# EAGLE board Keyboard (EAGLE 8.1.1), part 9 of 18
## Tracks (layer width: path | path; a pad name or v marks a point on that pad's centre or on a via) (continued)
S$8799 (continued)
  Bottom 0: 282.46,76.14 282.5,76.06
S$8800
  Bottom 0: 282.5,76.06 282.55,76.01
S$8801
  Bottom 0: 282.55,76.01 282.62,75.97
S$8802
  Bottom 0: 282.62,75.97 282.7,75.96
S$8803
  Bottom 0: 282.7,75.96 284.86,75.96
S$8804
  Bottom 0: 284.86,75.96 284.94,75.97
S$8805
  Bottom 0: 284.94,75.97 285.01,76.01
S$8806
  Bottom 0: 285.01,76.01 285.06,76.06
S$8807
  Bottom 0: 285.06,76.06 285.1,76.14
S$8808
  Bottom 0: 285.1,76.14 285.11,76.21
S$8809
  Bottom 0: 285.11,76.21 285.11,77.41
S$8810
  Bottom 0: 285.11,77.41 285.1,77.49
S$8811
  Bottom 0: 285.1,77.49 285.06,77.56
S$8812
  Bottom 0: 285.06,77.56 285.01,77.61
S$8813
  Bottom 0: 285.01,77.61 284.94,77.66
S$8814
  Bottom 0: 284.94,77.66 284.86,77.67
S$8815
  Bottom 0: 284.86,77.67 282.76,77.67
S$8816
  Bottom 0: 282.76,77.67 282.76,77.97
S$8817
  Bottom 0: 282.76,77.97 284.86,77.97
S$8818
  Bottom 0: 284.86,77.97 284.94,77.97
S$8819
  Bottom 0: 284.94,77.97 285.01,78.02
S$8820
  Bottom 0: 285.01,78.02 285.06,78.07
S$8821
  Bottom 0: 285.06,78.07 285.1,78.14
S$8822
  Bottom 0: 285.1,78.14 285.11,78.22
S$8823
  Bottom 0: 285.11,78.22 285.11,79.42
S$8824
  Bottom 0: 285.11,79.42 285.1,79.49
S$8825
  Bottom 0: 285.1,79.49 285.06,79.57
S$8826
  Bottom 0: 285.06,79.57 285.01,79.62
S$8827
  Bottom 0: 285.01,79.62 284.94,79.66
S$8828
  Bottom 0: 284.94,79.66 284.86,79.67
S$8829
  Bottom 0: 284.86,79.67 282.76,79.67
S$8830
  Bottom 0: 282.76,79.67 282.76,79.97
S$8831
  Bottom 0: 282.76,79.97 284.86,79.97
S$8832
  Bottom 0: 284.86,79.97 284.94,79.98
S$8833
  Bottom 0: 284.94,79.98 285.01,80.02
S$8834
  Bottom 0: 285.01,80.02 285.06,80.08
S$8835
  Bottom 0: 285.06,80.08 285.1,80.15
S$8836
  Bottom 0: 285.1,80.15 285.11,80.23
S$8837
  Bottom 0: 285.11,80.23 285.11,81.42
S$8838
  Bottom 0: 285.11,81.42 285.1,81.5
S$8839
  Bottom 0: 285.1,81.5 285.1,81.51
S$8840
  Bottom 0: 285.1,81.51 286.16,82.57
S$8841
  Bottom 0: 286.16,82.57 286.43,82.59
S$8842
  Bottom 0: 286.43,82.59 286.69,82.7
S$8843
  Bottom 0: 286.69,82.7 286.9,82.9
S$8844
  Bottom 0: 286.9,82.9 287.03,83.14
S$8845
  Bottom 0: 287.03,83.14 287.07,83.42
S$8846
  Bottom 0: 287.07,83.42 287.03,83.7
S$8847
  Bottom 0: 287.03,83.7 286.99,83.77
S$8848
  Bottom 0: 286.99,83.77 287.05,83.78
S$8849
  Bottom 0: 287.05,83.78 287.03,83.72
S$8850
  Bottom 0: 287.03,83.72 287.52,83.72
S$8851
  Bottom 0: 287.52,83.72 287.52,83.94
S$8852
  Bottom 0: 287.52,83.94 287.68,84.09
S$8853
  Bottom 0: 287.68,84.09 287.81,84.34
S$8854
  Bottom 0: 287.81,84.34 287.86,84.61
S$8855
  Bottom 0: 287.86,84.61 287.81,84.89
S$8856
  Bottom 0: 287.81,84.89 287.68,85.14
S$8857
  Bottom 0: 287.68,85.14 287.48,85.33
S$8858
  Bottom 0: 287.48,85.33 287.22,85.44
S$8859
  Bottom 0: 287.22,85.44 286.94,85.46
S$8860
  Bottom 0: 286.94,85.46 286.66,85.4
S$8861
  Bottom 0: 286.66,85.4 286.43,85.25
S$8862
  Bottom 0: 286.43,85.25 286.25,85.02
S$8863
  Bottom 0: 286.25,85.02 286.22,84.92
S$8864
  Bottom 0: 286.22,84.92 286.11,85.14
S$8865
  Bottom 0: 286.11,85.14 285.9,85.33
S$8866
  Bottom 0: 285.9,85.33 285.64,85.44
S$8867
  Bottom 0: 285.64,85.44 285.36,85.46
S$8868
  Bottom 0: 285.36,85.46 285.16,85.41
S$8869
  Bottom 0: 285.16,85.41 288.85,89.1
S$8870
  Bottom 0: 288.85,89.1 289.3,89.1
S$8871
  Bottom 0: 289.3,89.1 289.3,89.56
S$8872
  Bottom 0: 289.3,89.56 289.38,89.64
S$8873
  Bottom 0: 289.38,89.64 290.45,89.64
S$8874
  Bottom 0: 290.45,89.64 290.45,89.1
S$8875
  Bottom 0: 290.45,89.1 291.15,89.1
S$8876
  Bottom 0: 291.15,89.1 291.1,89.2
S$8877
  Bottom 0: 291.1,89.2 290.9,89.49
S$8878
  Bottom 0: 290.9,89.49 290.72,89.64
S$8879
  Bottom 0: 290.72,89.64 293.99,89.64
S$8880
  Bottom 0: 293.99,89.64 293.99,82.85
S$8881
  Bottom 0: 293.99,82.85 294,82.76
S$8882
  Bottom 0: 294,82.76 294.02,82.67
S$8883
  Bottom 0: 294.02,82.67 294.05,82.59
S$8884
  Bottom 0: 294.05,82.59 294.1,82.51
S$8885
  Bottom 0: 294.1,82.51 294.16,82.45
S$8886
  Bottom 0: 294.16,82.45 298.75,77.85
S$8887
  Bottom 0: 298.75,77.85 298.75,70.75
S$8888
  Bottom 0: 298.75,70.75 298.63,70.78
S$8889
  Bottom 0: 298.63,70.78 298.33,70.76
S$8890
  Bottom 0: 298.33,70.76 298.05,70.65
S$8891
  Bottom 0: 298.05,70.65 297.81,70.46
S$8892
  Bottom 0: 297.81,70.46 297.8,70.44
S$8893
  Bottom 0: 297.8,70.44 297.8,70.66
S$8894
  Bottom 0: 297.8,70.66 297.79,70.74
S$8895
  Bottom 0: 297.79,70.74 297.75,70.81
S$8896
  Bottom 0: 297.75,70.81 297.69,70.86
S$8897
  Bottom 0: 297.69,70.86 297.62,70.9
S$8898
  Bottom 0: 297.62,70.9 297.54,70.91
S$8899
  Bottom 0: 297.54,70.91 296.47,70.91
S$8900
  Bottom 0: 296.47,70.91 296.47,71.04
S$8901
  Bottom 0: 296.47,71.04 296.45,71.1
S$8902
  Bottom 0: 296.45,71.1 296.45,71.16
S$8903
  Bottom 0: 296.45,71.16 296.42,71.21
S$8904
  Bottom 0: 296.42,71.21 296.4,71.26
S$8905
  Bottom 0: 296.4,71.26 296.38,71.3
S$8906
  Bottom 0: 296.38,71.3 296.34,71.36
S$8907
  Bottom 0: 296.34,71.36 295.29,72.4
S$8908
  Bottom 0: 295.29,72.4 295.31,72.42
S$8909
  Bottom 0: 295.31,72.42 295.44,72.72
S$8910
  Bottom 0: 295.44,72.72 295.49,73.04
S$8911
  Bottom 0: 295.49,73.04 295.44,73.36
S$8912
  Bottom 0: 295.44,73.36 295.31,73.66
S$8913
  Bottom 0: 295.31,73.66 295.11,73.92
S$8914
  Bottom 0: 295.11,73.92 294.84,74.11
S$8915
  Bottom 0: 294.84,74.11 294.53,74.21
S$8916
  Bottom 0: 294.53,74.21 294.21,74.23
S$8917
  Bottom 0: 294.21,74.23 293.89,74.17
S$8918
  Bottom 0: 293.89,74.17 293.6,74.02
S$8919
  Bottom 0: 293.6,74.02 293.38,73.8
S$8920
  Bottom 0: 293.38,73.8 293.38,73.89
S$8921
  Bottom 0: 293.38,73.89 293.82,74.33
S$8922
  Bottom 0: 293.82,74.33 293.89,74.3
S$8923
  Bottom 0: 293.89,74.3 294.21,74.23
S$8924
  Bottom 0: 294.21,74.23 294.53,74.25
S$8925
  Bottom 0: 294.53,74.25 294.84,74.36
S$8926
  Bottom 0: 294.84,74.36 295.11,74.55
S$8927
  Bottom 0: 295.11,74.55 295.31,74.8
S$8928
  Bottom 0: 295.31,74.8 295.44,75.1
S$8929
  Bottom 0: 295.44,75.1 295.49,75.42
S$8930
  Bottom 0: 295.49,75.42 295.44,75.74
S$8931
  Bottom 0: 295.44,75.74 295.31,76.04
S$8932
  Bottom 0: 295.31,76.04 295.11,76.29
S$8933
  Bottom 0: 295.11,76.29 294.84,76.48
S$8934
  Bottom 0: 294.84,76.48 294.53,76.59
S$8935
  Bottom 0: 294.53,76.59 294.21,76.61
S$8936
  Bottom 0: 294.21,76.61 293.9,76.54
S$8937
  Bottom 0: 293.9,76.54 294.04,76.69
S$8938
  Bottom 0: 294.04,76.69 297,76.69
S$8939
  Bottom 0: 297,76.69 297.07,76.69
S$8940
  Bottom 0: 297.07,76.69 297.14,76.7
S$8941
  Bottom 0: 297.14,76.7 297.2,76.73
S$8942
  Bottom 0: 297.2,76.73 297.26,76.77
S$8943
  Bottom 0: 297.26,76.77 297.32,76.81
S$8944
  Bottom 0: 297.32,76.81 297.53,77.03
S$8945
  Bottom 0: 297.53,77.03 297.63,77.02
S$8946
  Bottom 0: 297.63,77.02 297.88,77.08
S$8947
  Bottom 0: 297.88,77.08 298.08,77.23
S$8948
  Bottom 0: 298.08,77.23 298.21,77.45
S$8949
  Bottom 0: 298.21,77.45 298.26,77.7
S$8950
  Bottom 0: 298.26,77.7 298.21,77.94
S$8951
  Bottom 0: 298.21,77.94 298.08,78.16
S$8952
  Bottom 0: 298.08,78.16 297.88,78.31
S$8953
  Bottom 0: 297.88,78.31 297.63,78.38
S$8954
  Bottom 0: 297.63,78.38 297.39,78.36
S$8955
  Bottom 0: 297.39,78.36 297.16,78.25
S$8956
  Bottom 0: 297.16,78.25 296.99,78.06
S$8957
  Bottom 0: 296.99,78.06 296.9,77.82
S$8958
  Bottom 0: 296.9,77.82 296.9,77.65
S$8959
  Bottom 0: 296.9,77.65 296.82,77.57
S$8960
  Bottom 0: 296.82,77.57 296.36,77.57
S$8961
  Bottom 0: 296.36,77.57 296.53,77.71
S$8962
  Bottom 0: 296.53,77.71 296.74,77.99
S$8963
  Bottom 0: 296.74,77.99 296.86,78.32
S$8964
  Bottom 0: 296.86,78.32 296.91,78.66
S$8965
  Bottom 0: 296.91,78.66 296.86,79.01
S$8966
  Bottom 0: 296.86,79.01 296.74,79.33
S$8967
  Bottom 0: 296.74,79.33 296.53,79.62
S$8968
  Bottom 0: 296.53,79.62 296.25,79.84
S$8969
  Bottom 0: 296.25,79.84 295.94,79.99
S$8970
  Bottom 0: 295.94,79.99 295.6,80.05
S$8971
  Bottom 0: 295.6,80.05 295.25,80.03
S$8972
  Bottom 0: 295.25,80.03 295.14,80
S$8973
  Bottom 0: 295.14,80 294.84,80.05
S$8974
  Bottom 0: 294.84,80.05 294.49,80.03
S$8975
  Bottom 0: 294.49,80.03 294.15,79.93
S$8976
  Bottom 0: 294.15,79.93 293.86,79.74
S$8977
  Bottom 0: 293.86,79.74 293.62,79.48
S$8978
  Bottom 0: 293.62,79.48 293.45,79.17
S$8979
  Bottom 0: 293.45,79.17 293.43,79.1
S$8980
  Bottom 0: 293.43,79.1 293,79.1
S$8981
  Bottom 0: 293,79.1 292.93,79.1
S$8982
  Bottom 0: 292.93,79.1 292.87,79.08
S$8983
  Bottom 0: 292.87,79.08 292.8,79.06
S$8984
  Bottom 0: 292.8,79.06 292.74,79.02
S$8985
  Bottom 0: 292.74,79.02 292.69,78.98
S$8986
  Bottom 0: 292.69,78.98 287.71,74
S$8987
  Bottom 0: 287.71,74 287.46,74.05
S$8988
  Bottom 0: 287.46,74.05 287.15,74.03
S$8989
  Bottom 0: 287.15,74.03 286.88,73.92
S$8990
  Bottom 0: 286.88,73.92 286.69,73.78
S$8991
  Bottom 0: 286.69,73.78 286.69,79.34
S$8992
  Bottom 0: 286.69,79.34 287.06,79.71
S$8993
  Bottom 0: 287.06,79.71 287.15,79.67
S$8994
  Bottom 0: 287.15,79.67 287.46,79.65
S$8995
  Bottom 0: 287.46,79.65 287.75,79.72
S$8996
  Bottom 0: 287.75,79.72 288.02,79.87
S$8997
  Bottom 0: 288.02,79.87 288.22,80.09
S$8998
  Bottom 0: 288.22,80.09 288.35,80.36
S$8999
  Bottom 0: 288.35,80.36 288.4,80.66
S$9000
  Bottom 0: 288.4,80.66 288.35,80.96
S$9001
  Bottom 0: 288.35,80.96 288.22,81.24
S$9002
  Bottom 0: 288.22,81.24 288.02,81.45
S$9003
  Bottom 0: 288.02,81.45 287.75,81.61
S$9004
  Bottom 0: 287.75,81.61 287.46,81.67
S$9005
  Bottom 0: 287.46,81.67 287.15,81.65
S$9006
  Bottom 0: 287.15,81.65 286.88,81.54
S$9007
  Bottom 0: 286.88,81.54 286.64,81.35
S$9008
  Bottom 0: 286.64,81.35 286.47,81.11
S$9009
  Bottom 0: 286.47,81.11 286.38,80.81
S$9010
  Bottom 0: 286.38,80.81 286.38,80.51
S$9011
  Bottom 0: 286.38,80.51 286.43,80.34
S$9012
  Bottom 0: 286.43,80.34 285.94,79.84
S$9013
  Bottom 0: 285.94,79.84 285.89,79.79
S$9014
  Bottom 0: 285.89,79.79 285.85,79.73
S$9015
  Bottom 0: 285.85,79.73 285.83,79.67
S$9016
  Bottom 0: 285.83,79.67 285.81,79.6
S$9017
  Bottom 0: 285.81,79.6 285.81,79.53
S$9018
  Bottom 0: 285.81,79.53 285.81,65.56
S$9019
  Bottom 0: 285.81,65.56 285.32,65.07
S$9020
  Bottom 0: 285.32,65.07 285.09,65.05
S$9021
  Bottom 0: 285.09,65.05 284.86,64.94
S$9022
  Bottom 0: 284.86,64.94 284.69,64.75
S$9023
  Bottom 0: 284.69,64.75 284.6,64.52
S$9024
  Bottom 0: 284.6,64.52 284.6,64.27
S$9025
  Bottom 0: 284.6,64.27 284.69,64.03
S$9026
  Bottom 0: 284.69,64.03 284.86,63.84
S$9027
  Bottom 0: 284.86,63.84 285.09,63.73
S$9028
  Bottom 0: 285.09,63.73 285.33,63.71
S$9029
  Bottom 0: 285.33,63.71 285.58,63.78
S$9030
  Bottom 0: 285.58,63.78 285.78,63.93
S$9031
  Bottom 0: 285.78,63.93 285.92,64.14
S$9032
  Bottom 0: 285.92,64.14 285.96,64.39
S$9033
  Bottom 0: 285.96,64.39 285.95,64.45
S$9034
  Bottom 0: 285.95,64.45 286.56,65.06
S$9035
  Bottom 0: 286.56,65.06 286.6,65.12
S$9036
  Bottom 0: 286.6,65.12 286.65,65.18
S$9037
  Bottom 0: 286.65,65.18 286.67,65.24
S$9038
  Bottom 0: 286.67,65.24 286.69,65.31
S$9039
  Bottom 0: 286.69,65.31 286.69,65.38
S$9040
  Bottom 0: 286.69,65.38 286.69,72.3
S$9041
  Bottom 0: 286.69,72.3 286.88,72.16
S$9042
  Bottom 0: 286.88,72.16 287.15,72.05
S$9043
  Bottom 0: 287.15,72.05 287.46,72.03
S$9044
  Bottom 0: 287.46,72.03 287.75,72.1
S$9045
  Bottom 0: 287.75,72.1 288.02,72.25
S$9046
  Bottom 0: 288.02,72.25 288.22,72.47
S$9047
  Bottom 0: 288.22,72.47 288.35,72.74
S$9048
  Bottom 0: 288.35,72.74 288.4,73.04
S$9049
  Bottom 0: 288.4,73.04 288.35,73.34
S$9050
  Bottom 0: 288.35,73.34 288.34,73.37
S$9051
  Bottom 0: 288.34,73.37 293.19,78.22
S$9052
  Bottom 0: 293.19,78.22 293.43,78.22
S$9053
  Bottom 0: 293.43,78.22 293.45,78.15
S$9054
  Bottom 0: 293.45,78.15 293.62,77.84
S$9055
  Bottom 0: 293.62,77.84 293.86,77.58
S$9056
  Bottom 0: 293.86,77.58 293.89,77.57
S$9057
  Bottom 0: 293.89,77.57 293.85,77.57
S$9058
  Bottom 0: 293.85,77.57 293.78,77.56
S$9059
  Bottom 0: 293.78,77.56 293.71,77.55
S$9060
  Bottom 0: 293.71,77.55 293.65,77.52
S$9061
  Bottom 0: 293.65,77.52 293.59,77.48
S$9062
  Bottom 0: 293.59,77.48 293.54,77.44
S$9063
  Bottom 0: 293.54,77.44 290.09,74
S$9064
  Bottom 0: 290.09,74 289.84,74.05
S$9065
  Bottom 0: 289.84,74.05 289.54,74.03
S$9066
  Bottom 0: 289.54,74.03 289.26,73.92
S$9067
  Bottom 0: 289.26,73.92 289.02,73.73
S$9068
  Bottom 0: 289.02,73.73 288.85,73.48
S$9069
  Bottom 0: 288.85,73.48 288.76,73.19
S$9070
  Bottom 0: 288.76,73.19 288.76,72.89
S$9071
  Bottom 0: 288.76,72.89 288.85,72.6
S$9072
  Bottom 0: 288.85,72.6 289.02,72.35
S$9073
  Bottom 0: 289.02,72.35 289.26,72.16
S$9074
  Bottom 0: 289.26,72.16 289.54,72.05
S$9075
  Bottom 0: 289.54,72.05 289.84,72.03
S$9076
  Bottom 0: 289.84,72.03 290.14,72.1
S$9077
  Bottom 0: 290.14,72.1 290.4,72.25
S$9078
  Bottom 0: 290.4,72.25 290.6,72.47
S$9079
  Bottom 0: 290.6,72.47 290.74,72.74
S$9080
  Bottom 0: 290.74,72.74 290.78,73.04
S$9081
  Bottom 0: 290.78,73.04 290.74,73.34
S$9082
  Bottom 0: 290.74,73.34 290.72,73.37
S$9083
  Bottom 0: 290.72,73.37 293.17,75.82
S$9084
  Bottom 0: 293.17,75.82 293.11,75.58
S$9085
  Bottom 0: 293.11,75.58 293.11,75.26
S$9086
  Bottom 0: 293.11,75.26 293.19,74.94
S$9087
  Bottom 0: 293.19,74.94 292.63,74.38
S$9088
  Bottom 0: 292.63,74.38 292.58,74.33
S$9089
  Bottom 0: 292.58,74.33 292.55,74.27
S$9090
  Bottom 0: 292.55,74.27 292.51,74.21
S$9091
  Bottom 0: 292.51,74.21 292.5,74.14
S$9092
  Bottom 0: 292.5,74.14 292.49,74.07
S$9093
  Bottom 0: 292.49,74.07 292.49,70.52
S$9094
  Bottom 0: 292.49,70.52 292.5,70.45
S$9095
  Bottom 0: 292.5,70.45 292.51,70.38
S$9096
  Bottom 0: 292.51,70.38 292.54,70.32
S$9097
  Bottom 0: 292.54,70.32 292.58,70.26
S$9098
  Bottom 0: 292.58,70.26 292.62,70.2
S$9099
  Bottom 0: 292.62,70.2 294.75,68.08
S$9100
  Bottom 0: 294.75,68.08 294.81,68.03
S$9101
  Bottom 0: 294.81,68.03 294.87,67.99
S$9102
  Bottom 0: 294.87,67.99 294.93,67.97
S$9103
  Bottom 0: 294.93,67.97 294.99,67.95
S$9104
  Bottom 0: 294.99,67.95 295.06,67.95
S$9105
  Bottom 0: 295.06,67.95 299.75,67.95
S$9106
  Bottom 0: 299.75,67.95 299.82,67.95
S$9107
  Bottom 0: 299.82,67.95 299.89,67.97
S$9108
  Bottom 0: 299.89,67.97 299.95,67.99
S$9109
  Bottom 0: 299.95,67.99 300.01,68.03
S$9110
  Bottom 0: 300.01,68.03 300.06,68.08
S$9111
  Bottom 0: 300.06,68.08 300.91,68.91
S$9112
  Bottom 0: 300.91,68.91 300.95,68.97
S$9113
  Bottom 0: 300.95,68.97 300.99,69.03
S$9114
  Bottom 0: 300.99,69.03 301.01,69.09
S$9115
  Bottom 0: 301.01,69.09 301.03,69.16
S$9116
  Bottom 0: 301.03,69.16 301.03,69.22
S$9117
  Bottom 0: 301.03,69.22 301.03,72.25
S$9118
  Bottom 0: 301.03,72.25 301.22,72.07
S$9119
  Bottom 0: 301.22,72.07 301.51,71.92
S$9120
  Bottom 0: 301.51,71.92 301.83,71.85
S$9121
  Bottom 0: 301.83,71.85 302.15,71.87
S$9122
  Bottom 0: 302.15,71.87 302.46,71.98
S$9123
  Bottom 0: 302.46,71.98 302.73,72.17
S$9124
  Bottom 0: 302.73,72.17 302.93,72.42
S$9125
  Bottom 0: 302.93,72.42 303.06,72.72
S$9126
  Bottom 0: 303.06,72.72 303.11,73.04
S$9127
  Bottom 0: 303.11,73.04 303.06,73.36
S$9128
  Bottom 0: 303.06,73.36 302.93,73.66
S$9129
  Bottom 0: 302.93,73.66 302.73,73.92
S$9130
  Bottom 0: 302.73,73.92 302.48,74.09
S$9131
  Bottom 0: 302.48,74.09 302.48,74.37
S$9132
  Bottom 0: 302.48,74.37 302.73,74.55
S$9133
  Bottom 0: 302.73,74.55 302.93,74.8
S$9134
  Bottom 0: 302.93,74.8 303.06,75.1
S$9135
  Bottom 0: 303.06,75.1 303.11,75.42
S$9136
  Bottom 0: 303.11,75.42 303.06,75.74
S$9137
  Bottom 0: 303.06,75.74 302.93,76.04
S$9138
  Bottom 0: 302.93,76.04 302.73,76.29
S$9139
  Bottom 0: 302.73,76.29 302.46,76.48
S$9140
  Bottom 0: 302.46,76.48 302.15,76.59
S$9141
  Bottom 0: 302.15,76.59 301.83,76.61
S$9142
  Bottom 0: 301.83,76.61 301.51,76.54
S$9143
  Bottom 0: 301.51,76.54 301.22,76.4
S$9144
  Bottom 0: 301.22,76.4 301.03,76.22
S$9145
  Bottom 0: 301.03,76.22 301.03,78.99
S$9146
  Bottom 0: 301.03,78.99 301.03,79.06
S$9147
  Bottom 0: 301.03,79.06 301.01,79.12
S$9148
  Bottom 0: 301.01,79.12 300.98,79.19
S$9149
  Bottom 0: 300.98,79.19 300.95,79.25
S$9150
  Bottom 0: 300.95,79.25 300.9,79.3
S$9151
  Bottom 0: 300.9,79.3 300.03,80.17
S$9152
  Bottom 0: 300.03,80.17 300.03,80.32
S$9153
  Bottom 0: 300.03,80.32 300.21,80.12
S$9154
  Bottom 0: 300.21,80.12 300.5,79.94
S$9155
  Bottom 0: 300.5,79.94 300.83,79.83
S$9156
  Bottom 0: 300.83,79.83 301.19,79.81
S$9157
  Bottom 0: 301.19,79.81 301.49,79.86
S$9158
  Bottom 0: 301.49,79.86 301.6,79.83
S$9159
  Bottom 0: 301.6,79.83 301.95,79.81
S$9160
  Bottom 0: 301.95,79.81 302.29,79.87
S$9161
  Bottom 0: 302.29,79.87 302.47,79.96
S$9162
  Bottom 0: 302.47,79.96 303.93,78.5
S$9163
  Bottom 0: 303.93,78.5 303.93,54.37
S$9164
  Bottom 0: 303.93,54.37 303.68,54.24
S$9165
  Bottom 0: 303.68,54.24 303.45,54.02
S$9166
  Bottom 0: 303.45,54.02 303.27,53.75
S$9167
  Bottom 0: 303.27,53.75 303.19,53.43
S$9168
  Bottom 0: 303.19,53.43 303.19,53.11
S$9169
  Bottom 0: 303.19,53.11 303.27,52.79
S$9170
  Bottom 0: 303.27,52.79 303.45,52.52
S$9171
  Bottom 0: 303.45,52.52 303.68,52.3
S$9172
  Bottom 0: 303.68,52.3 303.97,52.15
S$9173
  Bottom 0: 303.97,52.15 304.29,52.08
S$9174
  Bottom 0: 304.29,52.08 304.62,52.1
S$9175
  Bottom 0: 304.62,52.1 304.92,52.21
S$9176
  Bottom 0: 304.92,52.21 305.18,52.4
S$9177
  Bottom 0: 305.18,52.4 305.39,52.65
S$9178
  Bottom 0: 305.39,52.65 305.52,52.95
S$9179
  Bottom 0: 305.52,52.95 305.56,53.27
S$9180
  Bottom 0: 305.56,53.27 305.52,53.59
S$9181
  Bottom 0: 305.52,53.59 305.39,53.89
S$9182
  Bottom 0: 305.39,53.89 305.18,54.15
S$9183
  Bottom 0: 305.18,54.15 304.92,54.33
S$9184
  Bottom 0: 304.92,54.33 304.81,54.37
S$9185
  Bottom 0: 304.81,54.37 304.81,78.69
S$9186
  Bottom 0: 304.81,78.69 304.81,78.76
S$9187
  Bottom 0: 304.81,78.76 304.79,78.83
S$9188
  Bottom 0: 304.79,78.83 304.76,78.89
S$9189
  Bottom 0: 304.76,78.89 304.73,78.95
S$9190
  Bottom 0: 304.73,78.95 304.69,79.01
S$9191
  Bottom 0: 304.69,79.01 303.11,80.59
S$9192
  Bottom 0: 303.11,80.59 303.21,80.86
S$9193
  Bottom 0: 303.21,80.86 303.26,81.2
S$9194
  Bottom 0: 303.26,81.2 303.21,81.55
S$9195
  Bottom 0: 303.21,81.55 303.09,81.87
S$9196
  Bottom 0: 303.09,81.87 302.88,82.16
S$9197
  Bottom 0: 302.88,82.16 302.61,82.38
S$9198
  Bottom 0: 302.61,82.38 302.29,82.53
S$9199
  Bottom 0: 302.29,82.53 301.95,82.59
S$9200
  Bottom 0: 301.95,82.59 301.6,82.57
S$9201
  Bottom 0: 301.6,82.57 301.49,82.54
S$9202
  Bottom 0: 301.49,82.54 301.19,82.59
S$9203
  Bottom 0: 301.19,82.59 300.9,82.58
S$9204
  Bottom 0: 300.9,82.58 300.92,82.63
S$9205
  Bottom 0: 300.92,82.63 300.94,82.7
S$9206
  Bottom 0: 300.94,82.7 300.94,82.77
S$9207
  Bottom 0: 300.94,82.77 300.94,85.1
S$9208
  Bottom 0: 300.94,85.1 300.94,85.17
S$9209
  Bottom 0: 300.94,85.17 300.92,85.24
S$9210
  Bottom 0: 300.92,85.24 300.9,85.3
S$9211
  Bottom 0: 300.9,85.3 300.86,85.36
S$9212
  Bottom 0: 300.86,85.36 300.81,85.42
S$9213
  Bottom 0: 300.81,85.42 298.41,87.83
S$9214
  Bottom 0: 298.41,87.83 298.63,87.81
S$9215
  Bottom 0: 298.63,87.81 298.76,87.84
S$9216
  Bottom 0: 298.76,87.84 298.85,87.78
S$9217
  Bottom 0: 298.85,87.78 299.16,87.69
S$9218
  Bottom 0: 299.16,87.69 299.48,87.69
S$9219
  Bottom 0: 299.48,87.69 299.79,87.78
S$9220
  Bottom 0: 299.79,87.78 300.06,87.96
S$9221
  Bottom 0: 300.06,87.96 300.28,88.2
S$9222
  Bottom 0: 300.28,88.2 300.42,88.5
S$9223
  Bottom 0: 300.42,88.5 300.46,88.82
S$9224
  Bottom 0: 300.46,88.82 300.42,89.12
S$9225
  Bottom 0: 300.42,89.12 300.94,89.64
S$9226
  Bottom 0: 300.94,89.64 313.93,89.64
S$9227
  Bottom 0: 313.93,89.64 313.93,87.93
S$9228
  Bottom 0: 313.93,87.93 313.94,87.86
S$9229
  Bottom 0: 313.94,87.86 313.98,87.78
S$9230
  Bottom 0: 313.98,87.78 314.04,87.73
S$9231
  Bottom 0: 314.04,87.73 314.11,87.69
S$9232
  Bottom 0: 314.11,87.69 314.19,87.68
S$9233
  Bottom 0: 314.19,87.68 314.58,87.68
S$9234
  Bottom 0: 314.58,87.68 311.98,85.08
S$9235
  Bottom 0: 311.98,85.08 311.93,85.03
S$9236
  Bottom 0: 311.93,85.03 311.89,84.97
S$9237
  Bottom 0: 311.89,84.97 311.86,84.91
S$9238
  Bottom 0: 311.86,84.91 311.85,84.84
S$9239
  Bottom 0: 311.85,84.84 311.84,84.77
S$9240
  Bottom 0: 311.84,84.77 311.84,76.47
S$9241
  Bottom 0: 311.84,76.47 311.85,76.4
S$9242
  Bottom 0: 311.85,76.4 311.86,76.33
S$9243
  Bottom 0: 311.86,76.33 311.89,76.27
S$9244
  Bottom 0: 311.89,76.27 311.93,76.21
S$9245
  Bottom 0: 311.93,76.21 311.97,76.16
S$9246
  Bottom 0: 311.97,76.16 312.25,75.88
S$9247
  Bottom 0: 312.25,75.88 312.16,75.58
S$9248
  Bottom 0: 312.16,75.58 312.16,75.25
S$9249
  Bottom 0: 312.16,75.25 312.25,74.94
S$9250
  Bottom 0: 312.25,74.94 312.42,74.66
S$9251
  Bottom 0: 312.42,74.66 312.65,74.44
S$9252
  Bottom 0: 312.65,74.44 312.94,74.29
S$9253
  Bottom 0: 312.94,74.29 313.25,74.23
S$9254
  Bottom 0: 313.25,74.23 312.94,74.17
S$9255
  Bottom 0: 312.94,74.17 312.65,74.02
S$9256
  Bottom 0: 312.65,74.02 312.42,73.8
S$9257
  Bottom 0: 312.42,73.8 312.25,73.52
S$9258
  Bottom 0: 312.25,73.52 312.16,73.2
S$9259
  Bottom 0: 312.16,73.2 312.16,72.88
S$9260
  Bottom 0: 312.16,72.88 312.25,72.56
S$9261
  Bottom 0: 312.25,72.56 312.42,72.29
S$9262
  Bottom 0: 312.42,72.29 312.65,72.07
S$9263
  Bottom 0: 312.65,72.07 312.94,71.92
S$9264
  Bottom 0: 312.94,71.92 313.26,71.85
S$9265
  Bottom 0: 313.26,71.85 313.58,71.87
S$9266
  Bottom 0: 313.58,71.87 313.61,71.88
S$9267
  Bottom 0: 313.61,71.88 314.57,70.91
S$9268
  Bottom 0: 314.57,70.91 314.19,70.91
S$9269
  Bottom 0: 314.19,70.91 314.11,70.9
S$9270
  Bottom 0: 314.11,70.9 314.04,70.86
S$9271
  Bottom 0: 314.04,70.86 313.98,70.81
S$9272
  Bottom 0: 313.98,70.81 313.94,70.74
S$9273
  Bottom 0: 313.94,70.74 313.93,70.66
S$9274
  Bottom 0: 313.93,70.66 313.93,68.88
S$9275
  Bottom 0: 313.93,68.88 313.94,68.85
S$9276
  Bottom 0: 313.94,68.85 311.76,68.85
S$9277
  Bottom 0: 311.76,68.85 309.75,70.86
S$9278
  Bottom 0: 309.75,70.86 309.69,70.9
S$9279
  Bottom 0: 309.69,70.9 309.63,70.94
S$9280
  Bottom 0: 309.63,70.94 309.57,70.97
S$9281
  Bottom 0: 309.57,70.97 309.51,70.98
S$9282
  Bottom 0: 309.51,70.98 309.44,70.98
S$9283
  Bottom 0: 309.44,70.98 306.85,70.98
S$9284
  Bottom 0: 306.85,70.98 306.78,70.98
S$9285
  Bottom 0: 306.78,70.98 306.71,70.97
S$9286
  Bottom 0: 306.71,70.97 306.65,70.94
S$9287
  Bottom 0: 306.65,70.94 306.59,70.9
S$9288
  Bottom 0: 306.59,70.9 306.54,70.86
S$9289
  Bottom 0: 306.54,70.86 305.6,69.92
S$9290
  Bottom 0: 305.6,69.92 305.55,69.86
S$9291
  Bottom 0: 305.55,69.86 305.51,69.8
S$9292
  Bottom 0: 305.51,69.8 305.49,69.74
S$9293
  Bottom 0: 305.49,69.74 305.47,69.67
S$9294
  Bottom 0: 305.47,69.67 305.47,69.6
S$9295
  Bottom 0: 305.47,69.6 305.47,54.27
S$9296
  Bottom 0: 305.47,54.27 305.47,54.2
S$9297
  Bottom 0: 305.47,54.2 305.49,54.13
S$9298
  Bottom 0: 305.49,54.13 305.51,54.07
S$9299
  Bottom 0: 305.51,54.07 305.55,54.01
S$9300
  Bottom 0: 305.55,54.01 305.6,53.96
S$9301
  Bottom 0: 305.6,53.96 305.81,53.74
S$9302
  Bottom 0: 305.81,53.74 305.73,53.43
S$9303
  Bottom 0: 305.73,53.43 305.73,53.11
S$9304
  Bottom 0: 305.73,53.11 305.81,52.79
S$9305
  Bottom 0: 305.81,52.79 305.99,52.52
S$9306
  Bottom 0: 305.99,52.52 306.22,52.3
S$9307
  Bottom 0: 306.22,52.3 306.51,52.15
S$9308
  Bottom 0: 306.51,52.15 306.83,52.08
S$9309
  Bottom 0: 306.83,52.08 307.15,52.1
S$9310
  Bottom 0: 307.15,52.1 307.46,52.21
S$9311
  Bottom 0: 307.46,52.21 307.72,52.4
S$9312
  Bottom 0: 307.72,52.4 307.93,52.65
S$9313
  Bottom 0: 307.93,52.65 308.06,52.95
S$9314
  Bottom 0: 308.06,52.95 308.11,53.27
S$9315
  Bottom 0: 308.11,53.27 308.06,53.59
S$9316
  Bottom 0: 308.06,53.59 307.93,53.89
S$9317
  Bottom 0: 307.93,53.89 307.72,54.15
S$9318
  Bottom 0: 307.72,54.15 307.46,54.33
S$9319
  Bottom 0: 307.46,54.33 307.15,54.44
S$9320
  Bottom 0: 307.15,54.44 306.83,54.46
S$9321
  Bottom 0: 306.83,54.46 306.51,54.39
S$9322
  Bottom 0: 306.51,54.39 306.45,54.36
S$9323
  Bottom 0: 306.45,54.36 306.35,54.46
S$9324
  Bottom 0: 306.35,54.46 306.35,66.65
S$9325
  Bottom 0: 306.35,66.65 306.52,66.56
S$9326
  Bottom 0: 306.52,66.56 306.77,66.54
S$9327
  Bottom 0: 306.77,66.54 307.02,66.61
S$9328
  Bottom 0: 307.02,66.61 307.22,66.76
S$9329
  Bottom 0: 307.22,66.76 307.35,66.97
S$9330
  Bottom 0: 307.35,66.97 307.4,67.22
S$9331
  Bottom 0: 307.4,67.22 307.35,67.47
S$9332
  Bottom 0: 307.35,67.47 307.22,67.68
S$9333
  Bottom 0: 307.22,67.68 307.02,67.83
S$9334
  Bottom 0: 307.02,67.83 306.91,67.87
S$9335
  Bottom 0: 306.91,67.87 306.91,68.03
S$9336
  Bottom 0: 306.91,68.03 307.12,67.87
S$9337
  Bottom 0: 307.12,67.87 307.4,67.76
S$9338
  Bottom 0: 307.4,67.76 307.7,67.74
S$9339
  Bottom 0: 307.7,67.74 307.95,67.8
S$9340
  Bottom 0: 307.95,67.8 308.77,66.97
S$9341
  Bottom 0: 308.77,66.97 308.77,61.02
S$9342
  Bottom 0: 308.77,61.02 308.78,60.95
S$9343
  Bottom 0: 308.78,60.95 308.8,60.89
S$9344
  Bottom 0: 308.8,60.89 308.82,60.83
S$9345
  Bottom 0: 308.82,60.83 308.86,60.76
S$9346
  Bottom 0: 308.86,60.76 308.9,60.71
S$9347
  Bottom 0: 308.9,60.71 309.33,60.29
S$9348
  Bottom 0: 309.33,60.29 309.17,60.27
S$9349
  Bottom 0: 309.17,60.27 309.13,60.26
S$9350
  Bottom 0: 309.13,60.26 308.58,60.8
S$9351
  Bottom 0: 308.58,60.8 308.6,60.83
S$9352
  Bottom 0: 308.6,60.83 308.64,61.13
S$9353
  Bottom 0: 308.64,61.13 308.6,61.43
S$9354
  Bottom 0: 308.6,61.43 308.46,61.7
S$9355
  Bottom 0: 308.46,61.7 308.26,61.92
S$9356
  Bottom 0: 308.26,61.92 308,62.08
S$9357
  Bottom 0: 308,62.08 307.7,62.14
S$9358
  Bottom 0: 307.7,62.14 307.4,62.12
S$9359
  Bottom 0: 307.4,62.12 307.12,62.01
S$9360
  Bottom 0: 307.12,62.01 306.88,61.82
S$9361
  Bottom 0: 306.88,61.82 306.71,61.57
S$9362
  Bottom 0: 306.71,61.57 306.62,61.28
S$9363
  Bottom 0: 306.62,61.28 306.62,60.98
S$9364
  Bottom 0: 306.62,60.98 306.71,60.69
S$9365
  Bottom 0: 306.71,60.69 306.88,60.44
S$9366
  Bottom 0: 306.88,60.44 307.12,60.25
S$9367
  Bottom 0: 307.12,60.25 307.4,60.14
S$9368
  Bottom 0: 307.4,60.14 307.7,60.12
S$9369
  Bottom 0: 307.7,60.12 307.95,60.17
S$9370
  Bottom 0: 307.95,60.17 308.7,59.43
S$9371
  Bottom 0: 308.7,59.43 308.77,59.25
S$9372
  Bottom 0: 308.77,59.25 308.94,59.06
S$9373
  Bottom 0: 308.94,59.06 309.17,58.95
S$9374
  Bottom 0: 309.17,58.95 309.42,58.93
S$9375
  Bottom 0: 309.42,58.93 309.66,59
S$9376
  Bottom 0: 309.66,59 309.86,59.15
S$9377
  Bottom 0: 309.86,59.15 309.99,59.36
S$9378
  Bottom 0: 309.99,59.36 310.03,59.58
S$9379
  Bottom 0: 310.03,59.58 315.46,54.15
S$9380
  Bottom 0: 315.46,54.15 315.46,54
S$9381
  Bottom 0: 315.46,54 315.34,54.15
S$9382
  Bottom 0: 315.34,54.15 315.08,54.33
S$9383
  Bottom 0: 315.08,54.33 314.77,54.44
S$9384
  Bottom 0: 314.77,54.44 314.45,54.46
S$9385
  Bottom 0: 314.45,54.46 314.13,54.39
S$9386
  Bottom 0: 314.13,54.39 313.84,54.24
S$9387
  Bottom 0: 313.84,54.24 313.61,54.02
S$9388
  Bottom 0: 313.61,54.02 313.43,53.75
S$9389
  Bottom 0: 313.43,53.75 313.35,53.43
S$9390
  Bottom 0: 313.35,53.43 313.35,53.11
S$9391
  Bottom 0: 313.35,53.11 313.43,52.79
S$9392
  Bottom 0: 313.43,52.79 313.61,52.52
S$9393
  Bottom 0: 313.61,52.52 313.84,52.3
S$9394
  Bottom 0: 313.84,52.3 314.13,52.15
S$9395
  Bottom 0: 314.13,52.15 314.45,52.08
S$9396
  Bottom 0: 314.45,52.08 314.77,52.1
S$9397
  Bottom 0: 314.77,52.1 315.08,52.21
S$9398
  Bottom 0: 315.08,52.21 315.34,52.4
S$9399
  Bottom 0: 315.34,52.4 315.46,52.54
S$9400
  Bottom 0: 315.46,52.54 315.46,47.22
S$9401
  Bottom 0: 315.46,47.22 307.37,39.12
S$9402
  Bottom 0: 307.37,39.12 307.15,39.2
S$9403
  Bottom 0: 307.15,39.2 306.83,39.22
S$9404
  Bottom 0: 306.83,39.22 306.51,39.15
S$9405
  Bottom 0: 306.51,39.15 306.22,39.01
S$9406
  Bottom 0: 306.22,39.01 305.99,38.78
S$9407
  Bottom 0: 305.99,38.78 305.81,38.51
S$9408
  Bottom 0: 305.81,38.51 305.73,38.19
S$9409
  Bottom 0: 305.73,38.19 305.73,37.87
S$9410
  Bottom 0: 305.73,37.87 305.81,37.55
S$9411
  Bottom 0: 305.81,37.55 305.99,37.28
S$9412
  Bottom 0: 305.99,37.28 306.22,37.06
S$9413
  Bottom 0: 306.22,37.06 306.51,36.91
S$9414
  Bottom 0: 306.51,36.91 306.83,36.84
S$9415
  Bottom 0: 306.83,36.84 307.15,36.86
S$9416
  Bottom 0: 307.15,36.86 307.46,36.97
S$9417
  Bottom 0: 307.46,36.97 307.72,37.16
S$9418
  Bottom 0: 307.72,37.16 307.93,37.41
S$9419
  Bottom 0: 307.93,37.41 308.06,37.71
S$9420
  Bottom 0: 308.06,37.71 308.11,38.03
S$9421
  Bottom 0: 308.11,38.03 308.06,38.35
S$9422
  Bottom 0: 308.06,38.35 308,38.49
S$9423
  Bottom 0: 308,38.49 316.02,46.52
S$9424
  Bottom 0: 316.02,46.52 316.02,42.69
S$9425
  Bottom 0: 316.02,42.69 312.46,39.12
S$9426
  Bottom 0: 312.46,39.12 312.24,39.2
S$9427
  Bottom 0: 312.24,39.2 311.91,39.22
S$9428
  Bottom 0: 311.91,39.22 311.59,39.15
S$9429
  Bottom 0: 311.59,39.15 311.3,39.01
S$9430
  Bottom 0: 311.3,39.01 311.07,38.78
S$9431
  Bottom 0: 311.07,38.78 310.89,38.51
S$9432
  Bottom 0: 310.89,38.51 310.81,38.19
S$9433
  Bottom 0: 310.81,38.19 310.81,37.87
S$9434
  Bottom 0: 310.81,37.87 310.89,37.55
S$9435
  Bottom 0: 310.89,37.55 311.07,37.28
S$9436
  Bottom 0: 311.07,37.28 311.3,37.06
S$9437
  Bottom 0: 311.3,37.06 311.59,36.91
S$9438
  Bottom 0: 311.59,36.91 311.91,36.84
S$9439
  Bottom 0: 311.91,36.84 312.24,36.86
S$9440
  Bottom 0: 312.24,36.86 312.54,36.97
S$9441
  Bottom 0: 312.54,36.97 312.8,37.16
S$9442
  Bottom 0: 312.8,37.16 313.01,37.41
S$9443
  Bottom 0: 313.01,37.41 313.14,37.71
S$9444
  Bottom 0: 313.14,37.71 313.19,38.03
S$9445
  Bottom 0: 313.19,38.03 313.14,38.35
S$9446
  Bottom 0: 313.14,38.35 313.07,38.49
S$9447
  Bottom 0: 313.07,38.49 316.72,42.14
S$9448
  Bottom 0: 316.72,42.14 316.72,40.85
S$9449
  Bottom 0: 316.72,40.85 314.99,39.12
S$9450
  Bottom 0: 314.99,39.12 314.77,39.2
S$9451
  Bottom 0: 314.77,39.2 314.45,39.22
S$9452
  Bottom 0: 314.45,39.22 314.13,39.15
S$9453
  Bottom 0: 314.13,39.15 313.84,39.01
S$9454
  Bottom 0: 313.84,39.01 313.61,38.78
S$9455
  Bottom 0: 313.61,38.78 313.43,38.51
S$9456
  Bottom 0: 313.43,38.51 313.35,38.19
S$9457
  Bottom 0: 313.35,38.19 313.35,37.87
S$9458
  Bottom 0: 313.35,37.87 313.43,37.55
S$9459
  Bottom 0: 313.43,37.55 313.61,37.28
S$9460
  Bottom 0: 313.61,37.28 313.84,37.06
S$9461
  Bottom 0: 313.84,37.06 314.13,36.91
S$9462
  Bottom 0: 314.13,36.91 314.45,36.84
S$9463
  Bottom 0: 314.45,36.84 314.77,36.86
S$9464
  Bottom 0: 314.77,36.86 315.08,36.97
S$9465
  Bottom 0: 315.08,36.97 315.34,37.16
S$9466
  Bottom 0: 315.34,37.16 315.55,37.41
S$9467
  Bottom 0: 315.55,37.41 315.68,37.71
S$9468
  Bottom 0: 315.68,37.71 315.73,38.03
S$9469
  Bottom 0: 315.73,38.03 315.68,38.35
S$9470
  Bottom 0: 315.68,38.35 315.62,38.49
S$9471
  Bottom 0: 315.62,38.49 317.48,40.36
S$9472
  Bottom 0: 317.48,40.36 317.52,40.41
S$9473
  Bottom 0: 317.52,40.41 317.56,40.47
S$9474
  Bottom 0: 317.56,40.47 317.58,40.53
S$9475
  Bottom 0: 317.58,40.53 317.6,40.59
S$9476
  Bottom 0: 317.6,40.59 317.6,40.67
S$9477
  Bottom 0: 317.6,40.67 317.6,61.13
S$9478
  Bottom 0: 317.6,61.13 318.77,62.3
S$9479
  Bottom 0: 318.77,62.3 318.77,61.98
S$9480
  Bottom 0: 318.77,61.98 318.85,61.64
S$9481
  Bottom 0: 318.85,61.64 319.03,61.33
S$9482
  Bottom 0: 319.03,61.33 319.26,61.07
S$9483
  Bottom 0: 319.26,61.07 319.56,60.89
S$9484
  Bottom 0: 319.56,60.89 319.89,60.78
S$9485
  Bottom 0: 319.89,60.78 320.24,60.76
S$9486
  Bottom 0: 320.24,60.76 320.55,60.81
S$9487
  Bottom 0: 320.55,60.81 320.65,60.78
S$9488
  Bottom 0: 320.65,60.78 321,60.76
S$9489
  Bottom 0: 321,60.76 321.35,60.82
S$9490
  Bottom 0: 321.35,60.82 321.53,60.91
S$9491
  Bottom 0: 321.53,60.91 321.84,60.6
S$9492
  Bottom 0: 321.84,60.6 321.84,54.55
S$9493
  Bottom 0: 321.84,54.55 320.94,54.55
S$9494
  Bottom 0: 320.94,54.55 320.86,54.54
S$9495
  Bottom 0: 320.86,54.54 320.79,54.5
S$9496
  Bottom 0: 320.79,54.5 320.73,54.45
S$9497
  Bottom 0: 320.73,54.45 320.69,54.37
S$9498
  Bottom 0: 320.69,54.37 320.68,54.3
S$9499
  Bottom 0: 320.68,54.3 320.68,26.47
S$9500
  Bottom 0: 320.68,26.47 320.69,26.4
S$9501
  Bottom 0: 320.69,26.4 320.73,26.33
S$9502
  Bottom 0: 320.73,26.33 320.79,26.27
S$9503
  Bottom 0: 320.79,26.27 320.86,26.23
S$9504
  Bottom 0: 320.86,26.23 320.94,26.22
S$9505
  Bottom 0: 320.94,26.22 321.84,26.22
S$9506
  Bottom 0: 321.84,26.22 321.84,16.69
S$9507
  Bottom 0: 321.84,16.69 321.77,16.77
S$9508
  Bottom 0: 321.77,16.77 321.51,16.95
S$9509
  Bottom 0: 321.51,16.95 321.2,17.06
S$9510
  Bottom 0: 321.2,17.06 320.88,17.08
S$9511
  Bottom 0: 320.88,17.08 320.63,17.03
S$9512
  Bottom 0: 320.63,17.03 319.76,17.9
S$9513
  Bottom 0: 319.76,17.9 319.69,17.96
S$9514
  Bottom 0: 319.69,17.96 319.62,18.01
S$9515
  Bottom 0: 319.62,18.01 319.54,18.04
S$9516
  Bottom 0: 319.54,18.04 319.45,18.06
S$9517
  Bottom 0: 319.45,18.06 319.36,18.07
S$9518
  Bottom 0: 319.36,18.07 304.09,18.07
S$9519
  Bottom 0: 304.09,18.07 304.09,30
S$9520
  Bottom 0: 304.09,30 304.21,29.94
S$9521
  Bottom 0: 304.21,29.94 304.46,29.92
S$9522
  Bottom 0: 304.46,29.92 304.7,29.99
S$9523
  Bottom 0: 304.7,29.99 304.9,30.14
S$9524
  Bottom 0: 304.9,30.14 305.04,30.36
S$9525
  Bottom 0: 305.04,30.36 305.08,30.6
S$9526
  Bottom 0: 305.08,30.6 305.04,30.85
S$9527
  Bottom 0: 305.04,30.85 304.9,31.07
S$9528
  Bottom 0: 304.9,31.07 304.84,31.12
S$9529
  Bottom 0: 304.84,31.12 304.84,34.3
S$9530
  Bottom 0: 304.84,34.3 304.83,34.37
S$9531
  Bottom 0: 304.83,34.37 304.82,34.44
S$9532
  Bottom 0: 304.82,34.44 304.79,34.5
S$9533
  Bottom 0: 304.79,34.5 304.75,34.56
S$9534
  Bottom 0: 304.75,34.56 304.71,34.62
S$9535
  Bottom 0: 304.71,34.62 302.76,36.56
S$9536
  Bottom 0: 302.76,36.56 302.71,36.6
S$9537
  Bottom 0: 302.71,36.6 302.65,36.65
S$9538
  Bottom 0: 302.65,36.65 302.59,36.67
S$9539
  Bottom 0: 302.59,36.67 302.52,36.69
S$9540
  Bottom 0: 302.52,36.69 302.45,36.69
S$9541
  Bottom 0: 302.45,36.69 301.26,36.69
S$9542
  Bottom 0: 301.26,36.69 300.38,37.57
S$9543
  Bottom 0: 300.38,37.57 300.44,37.71
S$9544
  Bottom 0: 300.44,37.71 300.49,38.03
S$9545
  Bottom 0: 300.49,38.03 300.44,38.35
S$9546
  Bottom 0: 300.44,38.35 300.31,38.65
S$9547
  Bottom 0: 300.31,38.65 300.1,38.91
S$9548
  Bottom 0: 300.1,38.91 299.84,39.09
S$9549
  Bottom 0: 299.84,39.09 299.54,39.2
S$9550
  Bottom 0: 299.54,39.2 299.21,39.22
S$9551
  Bottom 0: 299.21,39.22 298.89,39.15
S$9552
  Bottom 0: 298.89,39.15 298.6,39.01
S$9553
  Bottom 0: 298.6,39.01 298.37,38.78
S$9554
  Bottom 0: 298.37,38.78 298.19,38.51
S$9555
  Bottom 0: 298.19,38.51 298.11,38.19
S$9556
  Bottom 0: 298.11,38.19 298.11,37.87
S$9557
  Bottom 0: 298.11,37.87 298.19,37.55
S$9558
  Bottom 0: 298.19,37.55 298.37,37.28
S$9559
  Bottom 0: 298.37,37.28 298.6,37.06
S$9560
  Bottom 0: 298.6,37.06 298.89,36.91
S$9561
  Bottom 0: 298.89,36.91 299.21,36.84
S$9562
  Bottom 0: 299.21,36.84 299.54,36.86
S$9563
  Bottom 0: 299.54,36.86 299.75,36.94
S$9564
  Bottom 0: 299.75,36.94 300.76,35.93
S$9565
  Bottom 0: 300.76,35.93 300.81,35.89
S$9566
  Bottom 0: 300.81,35.89 300.88,35.85
S$9567
  Bottom 0: 300.88,35.85 300.94,35.83
S$9568
  Bottom 0: 300.94,35.83 301,35.81
S$9569
  Bottom 0: 301,35.81 301.07,35.81
S$9570
  Bottom 0: 301.07,35.81 301.11,35.81
S$9571
  Bottom 0: 301.11,35.81 300.99,35.69
S$9572
  Bottom 0: 300.99,35.69 300.81,35.41
S$9573
  Bottom 0: 300.81,35.41 300.73,35.1
S$9574
  Bottom 0: 300.73,35.1 300.73,34.77
S$9575
  Bottom 0: 300.73,34.77 300.76,34.65
S$9576
  Bottom 0: 300.76,34.65 297.83,37.57
S$9577
  Bottom 0: 297.83,37.57 297.9,37.71
S$9578
  Bottom 0: 297.9,37.71 297.94,38.03
S$9579
  Bottom 0: 297.94,38.03 297.9,38.35
S$9580
  Bottom 0: 297.9,38.35 297.77,38.65
S$9581
  Bottom 0: 297.77,38.65 297.56,38.91
S$9582
  Bottom 0: 297.56,38.91 297.3,39.09
S$9583
  Bottom 0: 297.3,39.09 297,39.2
S$9584
  Bottom 0: 297,39.2 296.67,39.22
S$9585
  Bottom 0: 296.67,39.22 296.35,39.15
S$9586
  Bottom 0: 296.35,39.15 296.06,39.01
S$9587
  Bottom 0: 296.06,39.01 295.83,38.78
S$9588
  Bottom 0: 295.83,38.78 295.65,38.51
S$9589
  Bottom 0: 295.65,38.51 295.57,38.19
S$9590
  Bottom 0: 295.57,38.19 295.57,37.87
S$9591
  Bottom 0: 295.57,37.87 295.65,37.55
S$9592
  Bottom 0: 295.65,37.55 295.83,37.28
S$9593
  Bottom 0: 295.83,37.28 296.06,37.06
S$9594
  Bottom 0: 296.06,37.06 296.35,36.91
S$9595
  Bottom 0: 296.35,36.91 296.47,36.88
S$9596
  Bottom 0: 296.47,36.88 296.41,36.89
S$9597
  Bottom 0: 296.41,36.89 294.53,36.89
S$9598
  Bottom 0: 294.53,36.89 294.76,36.97
S$9599
  Bottom 0: 294.76,36.97 295.02,37.16
S$9600
  Bottom 0: 295.02,37.16 295.23,37.41
S$9601
  Bottom 0: 295.23,37.41 295.36,37.71
S$9602
  Bottom 0: 295.36,37.71 295.4,38.03
S$9603
  Bottom 0: 295.4,38.03 295.36,38.35
S$9604
  Bottom 0: 295.36,38.35 295.23,38.65
S$9605
  Bottom 0: 295.23,38.65 295.02,38.91
S$9606
  Bottom 0: 295.02,38.91 294.76,39.09
S$9607
  Bottom 0: 294.76,39.09 294.45,39.2
S$9608
  Bottom 0: 294.45,39.2 294.13,39.22
S$9609
  Bottom 0: 294.13,39.22 293.81,39.15
S$9610
  Bottom 0: 293.81,39.15 293.52,39.01
S$9611
  Bottom 0: 293.52,39.01 293.29,38.78
S$9612
  Bottom 0: 293.29,38.78 293.11,38.51
S$9613
  Bottom 0: 293.11,38.51 293.03,38.19
S$9614
  Bottom 0: 293.03,38.19 293.03,37.87
S$9615
  Bottom 0: 293.03,37.87 293.11,37.55
S$9616
  Bottom 0: 293.11,37.55 293.29,37.28
S$9617
  Bottom 0: 293.29,37.28 293.52,37.06
S$9618
  Bottom 0: 293.52,37.06 293.81,36.91
S$9619
  Bottom 0: 293.81,36.91 293.9,36.89
S$9620
  Bottom 0: 293.9,36.89 293.44,36.89
S$9621
  Bottom 0: 293.44,36.89 292.75,37.57
S$9622
  Bottom 0: 292.75,37.57 292.82,37.71
S$9623
  Bottom 0: 292.82,37.71 292.87,38.03
S$9624
  Bottom 0: 292.87,38.03 292.82,38.35
S$9625
  Bottom 0: 292.82,38.35 292.69,38.65
S$9626
  Bottom 0: 292.69,38.65 292.48,38.91
S$9627
  Bottom 0: 292.48,38.91 292.22,39.09
S$9628
  Bottom 0: 292.22,39.09 291.92,39.2
S$9629
  Bottom 0: 291.92,39.2 291.59,39.22
S$9630
  Bottom 0: 291.59,39.22 291.27,39.15
S$9631
  Bottom 0: 291.27,39.15 290.98,39.01
S$9632
  Bottom 0: 290.98,39.01 290.75,38.78
S$9633
  Bottom 0: 290.75,38.78 290.57,38.51
S$9634
  Bottom 0: 290.57,38.51 290.49,38.19
S$9635
  Bottom 0: 290.49,38.19 290.49,37.87
S$9636
  Bottom 0: 290.49,37.87 290.57,37.55
S$9637
  Bottom 0: 290.57,37.55 290.75,37.28
S$9638
  Bottom 0: 290.75,37.28 290.98,37.06
S$9639
  Bottom 0: 290.98,37.06 291.27,36.91
S$9640
  Bottom 0: 291.27,36.91 291.59,36.84
S$9641
  Bottom 0: 291.59,36.84 291.92,36.86
S$9642
  Bottom 0: 291.92,36.86 292.13,36.94
S$9643
  Bottom 0: 292.13,36.94 292.94,36.13
S$9644
  Bottom 0: 292.94,36.13 293,36.09
S$9645
  Bottom 0: 293,36.09 293.06,36.05
S$9646
  Bottom 0: 293.06,36.05 293.12,36.02
S$9647
  Bottom 0: 293.12,36.02 293.19,36.01
S$9648
  Bottom 0: 293.19,36.01 293.26,36.01
S$9649
  Bottom 0: 293.26,36.01 293.78,36.01
S$9650
  Bottom 0: 293.78,36.01 293.6,35.91
S$9651
  Bottom 0: 293.6,35.91 293.37,35.69
S$9652
  Bottom 0: 293.37,35.69 293.19,35.41
S$9653
  Bottom 0: 293.19,35.41 293.11,35.1
S$9654
  Bottom 0: 293.11,35.1 293.11,34.77
S$9655
  Bottom 0: 293.11,34.77 293.19,34.46
S$9656
  Bottom 0: 293.19,34.46 293.37,34.19
S$9657
  Bottom 0: 293.37,34.19 293.6,33.96
S$9658
  Bottom 0: 293.6,33.96 293.89,33.81
S$9659
  Bottom 0: 293.89,33.81 294.21,33.75
S$9660
  Bottom 0: 294.21,33.75 294.53,33.77
S$9661
  Bottom 0: 294.53,33.77 294.84,33.88
S$9662
  Bottom 0: 294.84,33.88 295.11,34.06
S$9663
  Bottom 0: 295.11,34.06 295.31,34.32
S$9664
  Bottom 0: 295.31,34.32 295.44,34.62
S$9665
  Bottom 0: 295.44,34.62 295.49,34.94
S$9666
  Bottom 0: 295.49,34.94 295.44,35.26
S$9667
  Bottom 0: 295.44,35.26 295.31,35.56
S$9668
  Bottom 0: 295.31,35.56 295.11,35.81
S$9669
  Bottom 0: 295.11,35.81 294.84,36
S$9670
  Bottom 0: 294.84,36 294.82,36.01
S$9671
  Bottom 0: 294.82,36.01 296.22,36.01
S$9672
  Bottom 0: 296.22,36.01 299.01,33.22
S$9673
  Bottom 0: 299.01,33.22 299.01,33.04
S$9674
  Bottom 0: 299.01,33.04 299.1,32.8
S$9675
  Bottom 0: 299.1,32.8 299.12,32.78
S$9676
  Bottom 0: 299.12,32.78 298.95,32.74
S$9677
  Bottom 0: 298.95,32.74 298.15,33.54
S$9678
  Bottom 0: 298.15,33.54 298.09,33.6
S$9679
  Bottom 0: 298.09,33.6 298.01,33.65
S$9680
  Bottom 0: 298.01,33.65 297.93,33.68
S$9681
  Bottom 0: 297.93,33.68 297.84,33.7
S$9682
  Bottom 0: 297.84,33.7 297.75,33.71
S$9683
  Bottom 0: 297.75,33.71 287.86,33.71
S$9684
  Bottom 0: 287.86,33.71 287.86,37.34
S$9685
  Bottom 0: 287.86,37.34 287.85,37.43
S$9686
  Bottom 0: 287.85,37.43 287.83,37.51
S$9687
  Bottom 0: 287.83,37.51 287.8,37.59
S$9688
  Bottom 0: 287.8,37.59 287.75,37.67
S$9689
  Bottom 0: 287.75,37.67 287.73,37.69
S$9690
  Bottom 0: 287.73,37.69 287.74,37.71
S$9691
  Bottom 0: 287.74,37.71 287.79,38.03
S$9692
  Bottom 0: 287.79,38.03 287.74,38.35
S$9693
  Bottom 0: 287.74,38.35 287.61,38.65
S$9694
  Bottom 0: 287.61,38.65 287.4,38.91
S$9695
  Bottom 0: 287.4,38.91 287.14,39.09
S$9696
  Bottom 0: 287.14,39.09 286.83,39.2
S$9697
  Bottom 0: 286.83,39.2 286.51,39.22
S$9698
  Bottom 0: 286.51,39.22 286.19,39.15
S$9699
  Bottom 0: 286.19,39.15 285.9,39.01
S$9700
  Bottom 0: 285.9,39.01 285.67,38.78
S$9701
  Bottom 0: 285.67,38.78 285.49,38.51
S$9702
  Bottom 0: 285.49,38.51 285.41,38.19
S$9703
  Bottom 0: 285.41,38.19 285.41,37.87
S$9704
  Bottom 0: 285.41,37.87 285.49,37.55
S$9705
  Bottom 0: 285.49,37.55 285.67,37.28
S$9706
  Bottom 0: 285.67,37.28 285.9,37.06
S$9707
  Bottom 0: 285.9,37.06 286.19,36.91
S$9708
  Bottom 0: 286.19,36.91 286.51,36.84
S$9709
  Bottom 0: 286.51,36.84 286.72,36.86
S$9710
  Bottom 0: 286.72,36.86 286.72,13.86
S$9711
  Bottom 0: 286.72,13.86 285.87,13.01
S$9712
  Bottom 0: 285.87,13.01 281.35,13.01
S$9713
  Bottom 0: 281.35,13.01 281.24,13.24
S$9714
  Bottom 0: 281.24,13.24 281.03,13.48
S$9715
  Bottom 0: 281.03,13.48 280.75,13.66
S$9716
  Bottom 0: 280.75,13.66 280.44,13.75
S$9717
  Bottom 0: 280.44,13.75 280.12,13.75
S$9718
  Bottom 0: 280.12,13.75 279.81,13.66
S$9719
  Bottom 0: 279.81,13.66 279.72,13.61
S$9720
  Bottom 0: 279.72,13.61 279.6,13.63
S$9721
  Bottom 0: 279.6,13.63 279.29,13.61
S$9722
  Bottom 0: 279.29,13.61 279.01,13.5
S$9723
  Bottom 0: 279.01,13.5 278.77,13.31
S$9724
  Bottom 0: 278.77,13.31 278.75,13.28
S$9725
  Bottom 0: 278.75,13.28 278.75,13.52
S$9726
  Bottom 0: 278.75,13.52 278.74,13.59
S$9727
  Bottom 0: 278.74,13.59 278.7,13.66
S$9728
  Bottom 0: 278.7,13.66 278.64,13.72
S$9729
  Bottom 0: 278.64,13.72 278.57,13.76
S$9730
  Bottom 0: 278.57,13.76 278.49,13.77
S$9731
  Bottom 0: 278.49,13.77 277.42,13.77
S$9732
  Bottom 0: 277.42,13.77 277.42,13.89
S$9733
  Bottom 0: 277.42,13.89 277.4,13.95
S$9734
  Bottom 0: 277.4,13.95 277.4,14.01
S$9735
  Bottom 0: 277.4,14.01 277.37,14.07
S$9736
  Bottom 0: 277.37,14.07 277.36,14.12
S$9737
  Bottom 0: 277.36,14.12 277.32,14.14
S$9738
  Bottom 0: 277.32,14.14 277.29,14.21
S$9739
  Bottom 0: 277.29,14.21 276.25,15.25
S$9740
  Bottom 0: 276.25,15.25 276.26,15.26
S$9741
  Bottom 0: 276.26,15.26 276.38,15.56
S$9742
  Bottom 0: 276.38,15.56 276.43,15.88
S$9743
  Bottom 0: 276.43,15.88 276.38,16.2
S$9744
  Bottom 0: 276.38,16.2 276.26,16.5
S$9745
  Bottom 0: 276.26,16.5 276.05,16.76
S$9746
  Bottom 0: 276.05,16.76 275.79,16.94
S$9747
  Bottom 0: 275.79,16.94 275.48,17.05
S$9748
  Bottom 0: 275.48,17.05 275.16,17.07
S$9749
  Bottom 0: 275.16,17.07 274.84,17
S$9750
  Bottom 0: 274.84,17 274.55,16.86
S$9751
  Bottom 0: 274.55,16.86 274.31,16.63
S$9752
  Bottom 0: 274.31,16.63 274.14,16.36
S$9753
  Bottom 0: 274.14,16.36 274.05,16.05
S$9754
  Bottom 0: 274.05,16.05 274.05,15.72
S$9755
  Bottom 0: 274.05,15.72 274.14,15.4
S$9756
  Bottom 0: 274.14,15.4 274.31,15.13
S$9757
  Bottom 0: 274.31,15.13 274.55,14.91
S$9758
  Bottom 0: 274.55,14.91 274.84,14.76
S$9759
  Bottom 0: 274.84,14.76 275.16,14.69
S$9760
  Bottom 0: 275.16,14.69 275.48,14.71
S$9761
  Bottom 0: 275.48,14.71 275.51,14.72
S$9762
  Bottom 0: 275.51,14.72 276.47,13.77
S$9763
  Bottom 0: 276.47,13.77 276.08,13.77
S$9764
  Bottom 0: 276.08,13.77 276.01,13.76
S$9765
  Bottom 0: 276.01,13.76 275.94,13.72
S$9766
  Bottom 0: 275.94,13.72 275.88,13.66
S$9767
  Bottom 0: 275.88,13.66 275.84,13.59
S$9768
  Bottom 0: 275.84,13.59 275.83,13.52
S$9769
  Bottom 0: 275.83,13.52 275.83,12.08
S$9770
  Bottom 0: 274.33,21.58 274.53,21.58
S$9771
  Bottom 0: 274.53,21.58 274.6,21.59
S$9772
  Bottom 0: 274.6,21.59 274.67,21.63
S$9773
  Bottom 0: 274.67,21.63 274.73,21.68
S$9774
  Bottom 0: 274.73,21.68 274.76,21.74
S$9775
  Bottom 0: 274.76,21.74 274.79,21.68
S$9776
  Bottom 0: 274.79,21.68 274.85,21.63
S$9777
  Bottom 0: 274.85,21.63 274.92,21.59
S$9778
  Bottom 0: 274.92,21.59 275,21.58
S$9779
  Bottom 0: 275,21.58 275.2,21.58
S$9780
  Bottom 0: 275.2,21.58 275.2,22.43
S$9781
  Bottom 0: 275.2,22.43 274.33,22.43
S$9782
  Bottom 0: 274.33,22.43 274.33,21.58
S$9783
  Bottom 0: 275.6,21.58 275.8,21.58
S$9784
  Bottom 0: 275.8,21.58 275.87,21.59
S$9785
  Bottom 0: 275.87,21.59 275.94,21.63
S$9786
  Bottom 0: 275.94,21.63 276,21.68
S$9787
  Bottom 0: 276,21.68 276.03,21.74
S$9788
  Bottom 0: 276.03,21.74 276.06,21.68
S$9789
  Bottom 0: 276.06,21.68 276.12,21.63
S$9790
  Bottom 0: 276.12,21.63 276.19,21.59
S$9791
  Bottom 0: 276.19,21.59 276.27,21.58
S$9792
  Bottom 0: 276.27,21.58 276.47,21.58
S$9793
  Bottom 0: 276.47,21.58 276.47,22.43
S$9794
  Bottom 0: 276.47,22.43 275.6,22.43
S$9795
  Bottom 0: 275.6,22.43 275.6,21.58
S$9796
  Bottom 0: 285.45,21.72 285.53,21.75
S$9797
  Bottom 0: 285.53,21.75 285.8,21.94
S$9798
  Bottom 0: 285.8,21.94 286.01,22.19
S$9799
  Bottom 0: 286.01,22.19 286.07,22.34
S$9800
  Bottom 0: 286.07,22.34 285.45,22.34
S$9801
  Bottom 0: 285.45,22.34 285.45,21.72
S$9802
  Bottom 0: 284.52,21.73 284.52,22.34
S$9803
  Bottom 0: 284.52,22.34 283.88,22.34
S$9804
  Bottom 0: 283.88,22.34 283.89,22.33
S$9805
  Bottom 0: 283.89,22.33 284.06,22.06
S$9806
  Bottom 0: 284.06,22.06 284.3,21.84
S$9807
  Bottom 0: 284.3,21.84 284.52,21.73
S$9808
  Bottom 0: 285.45,23.28 286.07,23.28
S$9809
  Bottom 0: 286.07,23.28 286.01,23.43
S$9810
  Bottom 0: 286.01,23.43 285.8,23.69
S$9811
  Bottom 0: 285.8,23.69 285.53,23.87
S$9812
  Bottom 0: 285.53,23.87 285.45,23.9
S$9813
  Bottom 0: 285.45,23.9 285.45,23.28
S$9814
  Bottom 0: 283.88,23.28 284.52,23.28
S$9815
  Bottom 0: 284.52,23.28 284.52,23.9
S$9816
  Bottom 0: 284.52,23.9 284.3,23.79
S$9817
  Bottom 0: 284.3,23.79 284.06,23.56
S$9818
  Bottom 0: 284.06,23.56 283.89,23.29
S$9819
  Bottom 0: 283.89,23.29 283.88,23.28
S$9820
  Bottom 0: 274.33,23.63 275.2,23.63
S$9821
  Bottom 0: 275.2,23.63 275.2,24.48
S$9822
  Bottom 0: 275.2,24.48 275,24.48
S$9823
  Bottom 0: 275,24.48 274.92,24.47
S$9824
  Bottom 0: 274.92,24.47 274.85,24.43
S$9825
  Bottom 0: 274.85,24.43 274.79,24.38
S$9826
  Bottom 0: 274.79,24.38 274.76,24.32
S$9827
  Bottom 0: 274.76,24.32 274.73,24.38
S$9828
  Bottom 0: 274.73,24.38 274.67,24.43
S$9829
  Bottom 0: 274.67,24.43 274.6,24.47
S$9830
  Bottom 0: 274.6,24.47 274.53,24.48
S$9831
  Bottom 0: 274.53,24.48 274.33,24.48
S$9832
  Bottom 0: 274.33,24.48 274.33,23.63
S$9833
  Bottom 0: 275.6,23.63 276.47,23.63
S$9834
  Bottom 0: 276.47,23.63 276.47,24.48
S$9835
  Bottom 0: 276.47,24.48 276.27,24.48
S$9836
  Bottom 0: 276.27,24.48 276.19,24.47
S$9837
  Bottom 0: 276.19,24.47 276.12,24.43
S$9838
  Bottom 0: 276.12,24.43 276.06,24.38
S$9839
  Bottom 0: 276.06,24.38 276.03,24.32
S$9840
  Bottom 0: 276.03,24.32 276,24.38
S$9841
  Bottom 0: 276,24.38 275.94,24.43
S$9842
  Bottom 0: 275.94,24.43 275.87,24.47
S$9843
  Bottom 0: 275.87,24.47 275.8,24.48
S$9844
  Bottom 0: 275.8,24.48 275.6,24.48
S$9845
  Bottom 0: 275.6,24.48 275.6,23.63
S$9846
  Bottom 0: 281.34,29.24 281.66,29.26
S$9847
  Bottom 0: 281.66,29.26 281.96,29.36
S$9848
  Bottom 0: 281.96,29.36 282.23,29.55
S$9849
  Bottom 0: 282.23,29.55 282.44,29.81
S$9850
  Bottom 0: 282.44,29.81 282.57,30.11
S$9851
  Bottom 0: 282.57,30.11 282.61,30.43
S$9852
  Bottom 0: 282.61,30.43 282.57,30.75
S$9853
  Bottom 0: 282.57,30.75 282.44,31.05
S$9854
  Bottom 0: 282.44,31.05 282.23,31.3
S$9855
  Bottom 0: 282.23,31.3 281.96,31.49
S$9856
  Bottom 0: 281.96,31.49 281.86,31.52
S$9857
  Bottom 0: 281.86,31.52 281.86,39.69
S$9858
  Bottom 0: 281.86,39.69 290.46,48.3
S$9859
  Bottom 0: 290.46,48.3 290.47,48.28
S$9860
  Bottom 0: 290.47,48.28 290.69,48.17
S$9861
  Bottom 0: 290.69,48.17 290.94,48.15
S$9862
  Bottom 0: 290.94,48.15 291.19,48.21
S$9863
  Bottom 0: 291.19,48.21 291.39,48.37
S$9864
  Bottom 0: 291.39,48.37 291.52,48.58
S$9865
  Bottom 0: 291.52,48.58 291.57,48.83
S$9866
  Bottom 0: 291.57,48.83 291.52,49.08
S$9867
  Bottom 0: 291.52,49.08 291.39,49.29
S$9868
  Bottom 0: 291.39,49.29 291.32,49.35
S$9869
  Bottom 0: 291.32,49.35 291.27,49.55
S$9870
  Bottom 0: 291.27,49.55 291.14,49.7
S$9871
  Bottom 0: 291.14,49.7 290.95,49.78
S$9872
  Bottom 0: 290.95,49.78 290.74,49.77
S$9873
  Bottom 0: 290.74,49.77 290.56,49.66
S$9874
  Bottom 0: 290.56,49.66 281.1,40.2
S$9875
  Bottom 0: 281.1,40.2 281.06,40.14
S$9876
  Bottom 0: 281.06,40.14 281.02,40.08
S$9877
  Bottom 0: 281.02,40.08 281,40.02
S$9878
  Bottom 0: 281,40.02 280.98,39.95
S$9879
  Bottom 0: 280.98,39.95 280.98,39.88
S$9880
  Bottom 0: 280.98,39.88 280.98,31.53
S$9881
  Bottom 0: 280.98,31.53 280.73,31.4
S$9882
  Bottom 0: 280.73,31.4 280.5,31.18
S$9883
  Bottom 0: 280.5,31.18 280.32,30.9
S$9884
  Bottom 0: 280.32,30.9 280.24,30.59
S$9885
  Bottom 0: 280.24,30.59 280.24,30.26
S$9886
  Bottom 0: 280.24,30.26 280.32,29.95
S$9887
  Bottom 0: 280.32,29.95 280.5,29.68
S$9888
  Bottom 0: 280.5,29.68 280.73,29.45
S$9889
  Bottom 0: 280.73,29.45 281.01,29.3
S$9890
  Bottom 0: 281.01,29.3 281.34,29.24
S$9891
  Bottom 0: 306.24,29.36 306.55,29.43
S$9892
  Bottom 0: 306.55,29.43 306.83,29.58
S$9893
  Bottom 0: 306.83,29.58 307.05,29.82
S$9894
  Bottom 0: 307.05,29.82 307.19,30.11
S$9895
  Bottom 0: 307.19,30.11 307.23,30.43
S$9896
  Bottom 0: 307.23,30.43 307.19,30.74
S$9897
  Bottom 0: 307.19,30.74 307.05,31.03
S$9898
  Bottom 0: 307.05,31.03 306.83,31.27
S$9899
  Bottom 0: 306.83,31.27 306.55,31.43
S$9900
  Bottom 0: 306.55,31.43 306.24,31.5
S$9901
  Bottom 0: 306.24,31.5 305.92,31.48
S$9902
  Bottom 0: 305.92,31.48 305.62,31.36
S$9903
  Bottom 0: 305.62,31.36 305.37,31.16
S$9904
  Bottom 0: 305.37,31.16 305.19,30.89
S$9905
  Bottom 0: 305.19,30.89 305.09,30.59
S$9906
  Bottom 0: 305.09,30.59 305.09,30.26
S$9907
  Bottom 0: 305.09,30.26 305.19,29.96
S$9908
  Bottom 0: 305.19,29.96 305.37,29.7
S$9909
  Bottom 0: 305.37,29.7 305.62,29.49
S$9910
  Bottom 0: 305.62,29.49 305.92,29.38
S$9911
  Bottom 0: 305.92,29.38 306.24,29.36
S$9912
  Bottom 0: 312.74,29.36 313.05,29.43
S$9913
  Bottom 0: 313.05,29.43 313.33,29.58
S$9914
  Bottom 0: 313.33,29.58 313.55,29.82
S$9915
